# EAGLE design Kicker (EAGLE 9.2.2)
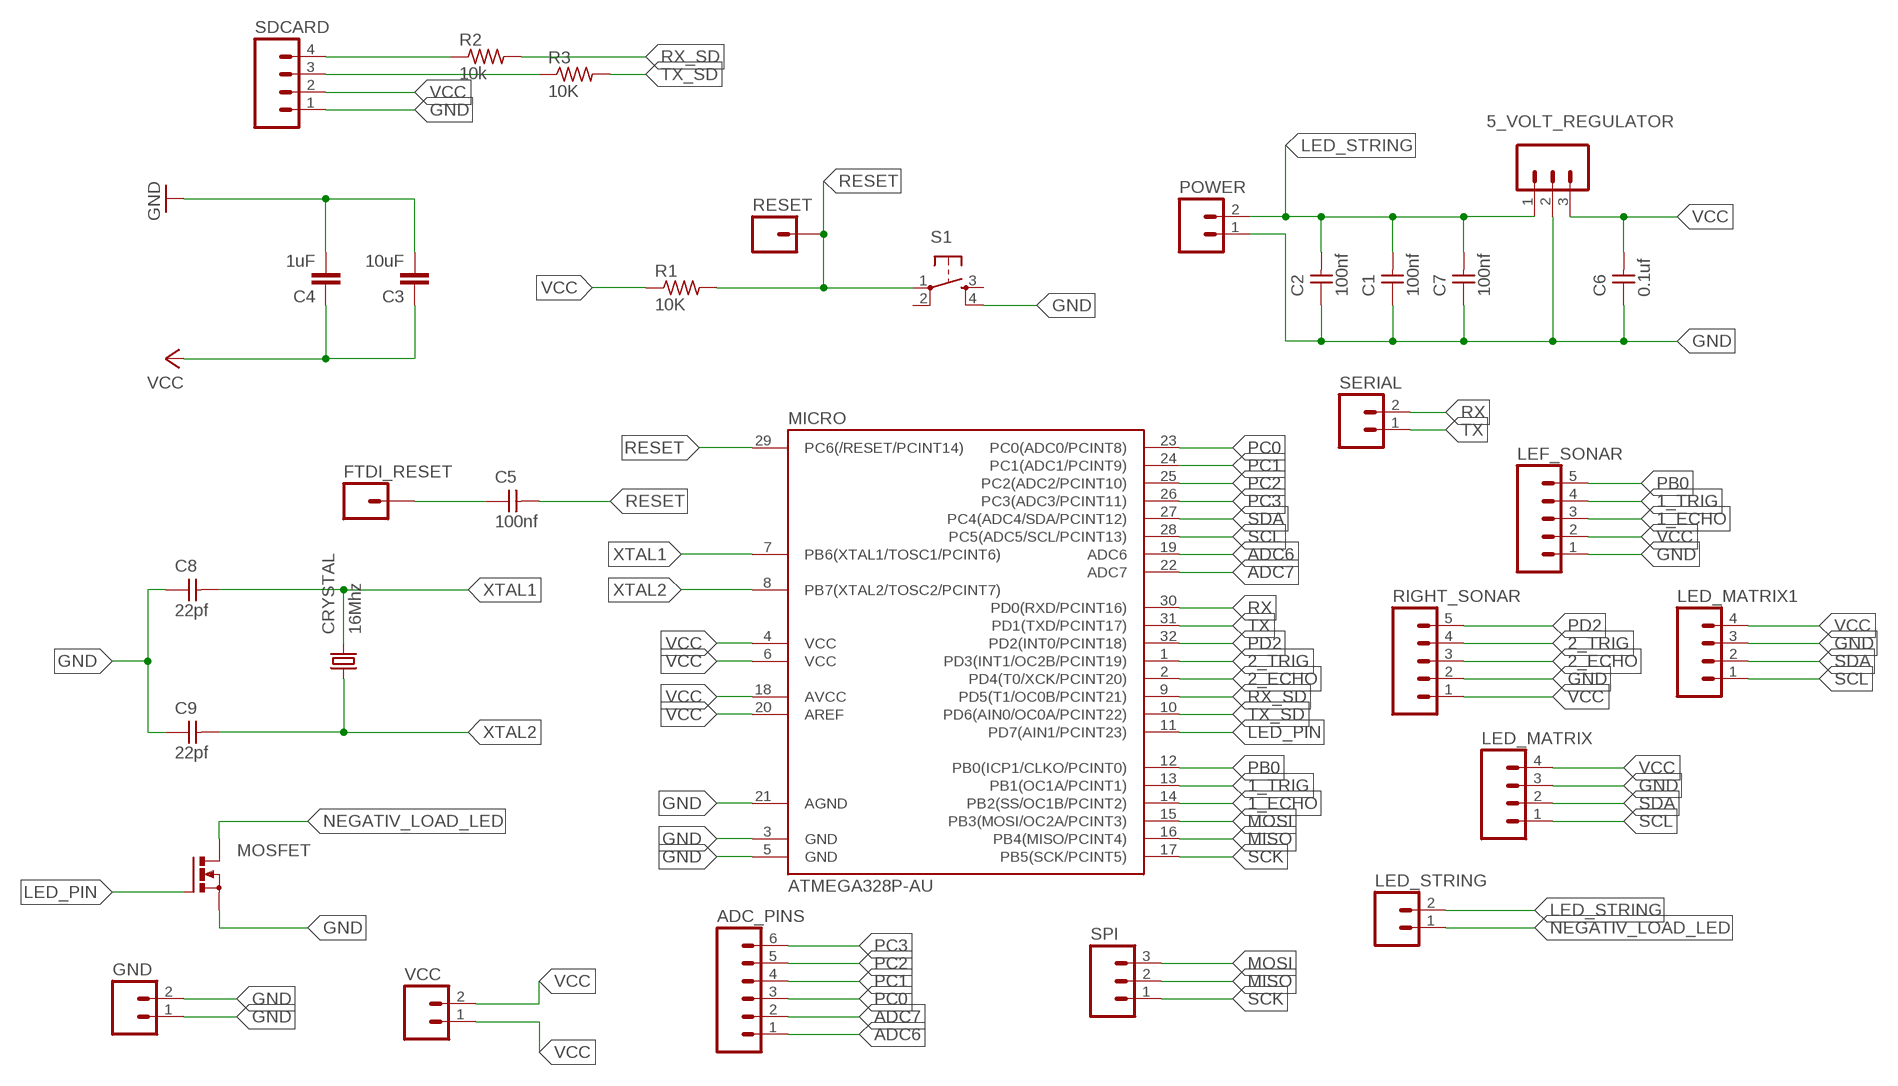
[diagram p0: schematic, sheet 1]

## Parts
5_VOLT_REGULATOR  M03  [03P]
ADC_PINS  M06  [06P]
C1  100nf  UNPOLARIZED_CAPACITOR1206  [1206]
C2  100nf  UNPOLARIZED_CAPACITOR1206  [1206]
C3  10uF  CAP1206  [1206]
C4  1uF  CAP1206  [1206]
C5  100nf  UNPOLARIZED_CAPACITOR1206  [1206]
C6  0.1uf  UNPOLARIZED_CAPACITOR1206  [1206]
C7  100nf  UNPOLARIZED_CAPACITOR1206  [1206]
C8  22pf  UNPOLARIZED_CAPACITOR1206  [1206]
C9  22pf  UNPOLARIZED_CAPACITOR1206  [1206]
CRYSTAL  16Mhz  KX-12B  [6.0X3.5_2]
FTDI_RESET  M01PTH  [1X01]
GND  M02  [02P]
LED_MATRIX  M04  [04P]
LED_MATRIX1  M04  [04P]
LED_STRING  M02  [02P]
LEF_SONAR  M05  [05P]
MICRO  ATMEGA328P-AU  ATMEGA48/88/168-AU  [TQFP32-08]
MOSFET  PMOSFET_NTO220BV  [TO220BV]
POWER  M02  [02P]
R1  10K  RESISTOR1206  [1206]
R2  10k  RESISTOR1206  [1206]
R3  10K  RESISTOR1206  [1206]
RESET  M01PTH  [1X01]
RIGHT_SONAR  M05  [05P]
S1  6MM_SWITCH6MM_SWITCH  [6MM_SWITCH]
SDCARD  M04  [04P]
SERIAL  M02  [02P]
SPI  M03  [03P]
VCC  M02  [02P]

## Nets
1_ECHO: LEF_SONAR.3 MICRO.14(PB2(SS/OC1B/PCINT2))
1_TRIG: LEF_SONAR.4 MICRO.13(PB1(OC1A/PCINT1))
2_ECHO: MICRO.2(PD4(T0/XCK/PCINT20)) RIGHT_SONAR.3
2_TRIG: MICRO.1(PD3(INT1/OC2B/PCINT19)) RIGHT_SONAR.4
ADC6: ADC_PINS.1 MICRO.19(ADC6)
ADC7: ADC_PINS.2 MICRO.22(ADC7)
GND: 5_VOLT_REGULATOR.2 C1.1 C2.1 C3.2 C4.2 C6.1 C7.1 C8.1 C9.1 GND.1 GND.2 LED_MATRIX1.3 LED_MATRIX.3 LEF_SONAR.1 MICRO.3(GND) MICRO.5(GND) MICRO.21(AGND) MOSFET.S POWER.1 RIGHT_SONAR.2 S1.4(S1) SDCARD.1
LED_PIN: MICRO.11(PD7(AIN1/PCINT23)) MOSFET.G
LED_STRING: 5_VOLT_REGULATOR.1 C1.2 C2.2 C7.2 LED_STRING.2 POWER.2
MISO: MICRO.16(PB4(MISO/PCINT4)) SPI.2
MOSI: MICRO.15(PB3(MOSI/OC2A/PCINT3)) SPI.3
N$2: R2.1 SDCARD.4
N$3: C5.1 FTDI_RESET.1
N$4: R3.1 SDCARD.3
NEGATIV_LOAD_LED: LED_STRING.1 MOSFET.D
PB0: LEF_SONAR.5 MICRO.12(PB0(ICP1/CLKO/PCINT0))
PC0: ADC_PINS.3 MICRO.23(PC0(ADC0/PCINT8))
PC1: ADC_PINS.4 MICRO.24(PC1(ADC1/PCINT9))
PC2: ADC_PINS.5 MICRO.25(PC2(ADC2/PCINT10))
PC3: ADC_PINS.6 MICRO.26(PC3(ADC3/PCINT11))
PD2: MICRO.32(PD2(INT0/PCINT18)) RIGHT_SONAR.5
RESET: C5.2 MICRO.29(PC6(/RESET/PCINT14)) R1.2 RESET.1 S1.1(P)
RX: MICRO.30(PD0(RXD/PCINT16)) SERIAL.2
RX_SD: MICRO.9(PD5(T1/OC0B/PCINT21)) R2.2
SCK: MICRO.17(PB5(SCK/PCINT5)) SPI.1
SCL: LED_MATRIX1.1 LED_MATRIX.1 MICRO.28(PC5(ADC5/SCL/PCINT13))
SDA: LED_MATRIX1.2 LED_MATRIX.2 MICRO.27(PC4(ADC4/SDA/PCINT12))
TX: MICRO.31(PD1(TXD/PCINT17)) SERIAL.1
TX_SD: MICRO.10(PD6(AIN0/OC0A/PCINT22)) R3.2
VCC: 5_VOLT_REGULATOR.3 C3.1 C4.1 C6.2 LED_MATRIX1.4 LED_MATRIX.4 LEF_SONAR.2 MICRO.4(VCC) MICRO.6(VCC) MICRO.18(AVCC) MICRO.20(AREF) R1.1 RIGHT_SONAR.1 SDCARD.2 VCC.1 VCC.2
XTAL1: C8.2 CRYSTAL.2 MICRO.7(PB6(XTAL1/TOSC1/PCINT6))
XTAL2: C9.2 CRYSTAL.1 MICRO.8(PB7(XTAL2/TOSC2/PCINT7))
Unconnected: S1.2(P1) S1.3(S)

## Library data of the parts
5_VOLT_REGULATOR SPI = con-amp-quick:M03: AMP QUICK CONNECTOR; OC_FARNELL: unknown; OC_NEWARK: unknown
ADC_PINS = con-amp-quick:M06: AMP QUICK CONNECTOR; OC_FARNELL: unknown; OC_NEWARK: unknown
C1 C2 C5-C9 = FAB_Hello:UNPOLARIZED_CAPACITOR: unpolarized_capacitor
C3 C4 = 01_SparkFun:CAP: Capacitor
CRYSTAL = crystal-geyer_V1_0:KX
FTDI_RESET RESET = flight_controller.lbr01_SparkFun:M01: Header 1
GND LED_STRING POWER SERIAL VCC = con-amp-quick:M02: AMP QUICK CONNECTOR; OC_FARNELL: unknown; OC_NEWARK: unknown
LED_MATRIX LED_MATRIX1 SDCARD = con-amp-quick:M04: AMP QUICK CONNECTOR; OC_FARNELL: unknown; OC_NEWARK: unknown
LEF_SONAR RIGHT_SONAR = con-amp-quick:M05: AMP QUICK CONNECTOR; OC_FARNELL: unknown; OC_NEWARK: unknown
MICRO = atmega8:ATMEGA48/88/168
MOSFET = transistor-power:PMOSFET_N: Power MOSFET N-Channel
R1-R3 = FAB_Hello:RESISTOR
S1 = FAB_Hello:6MM_SWITCH: OMRON SWITCH

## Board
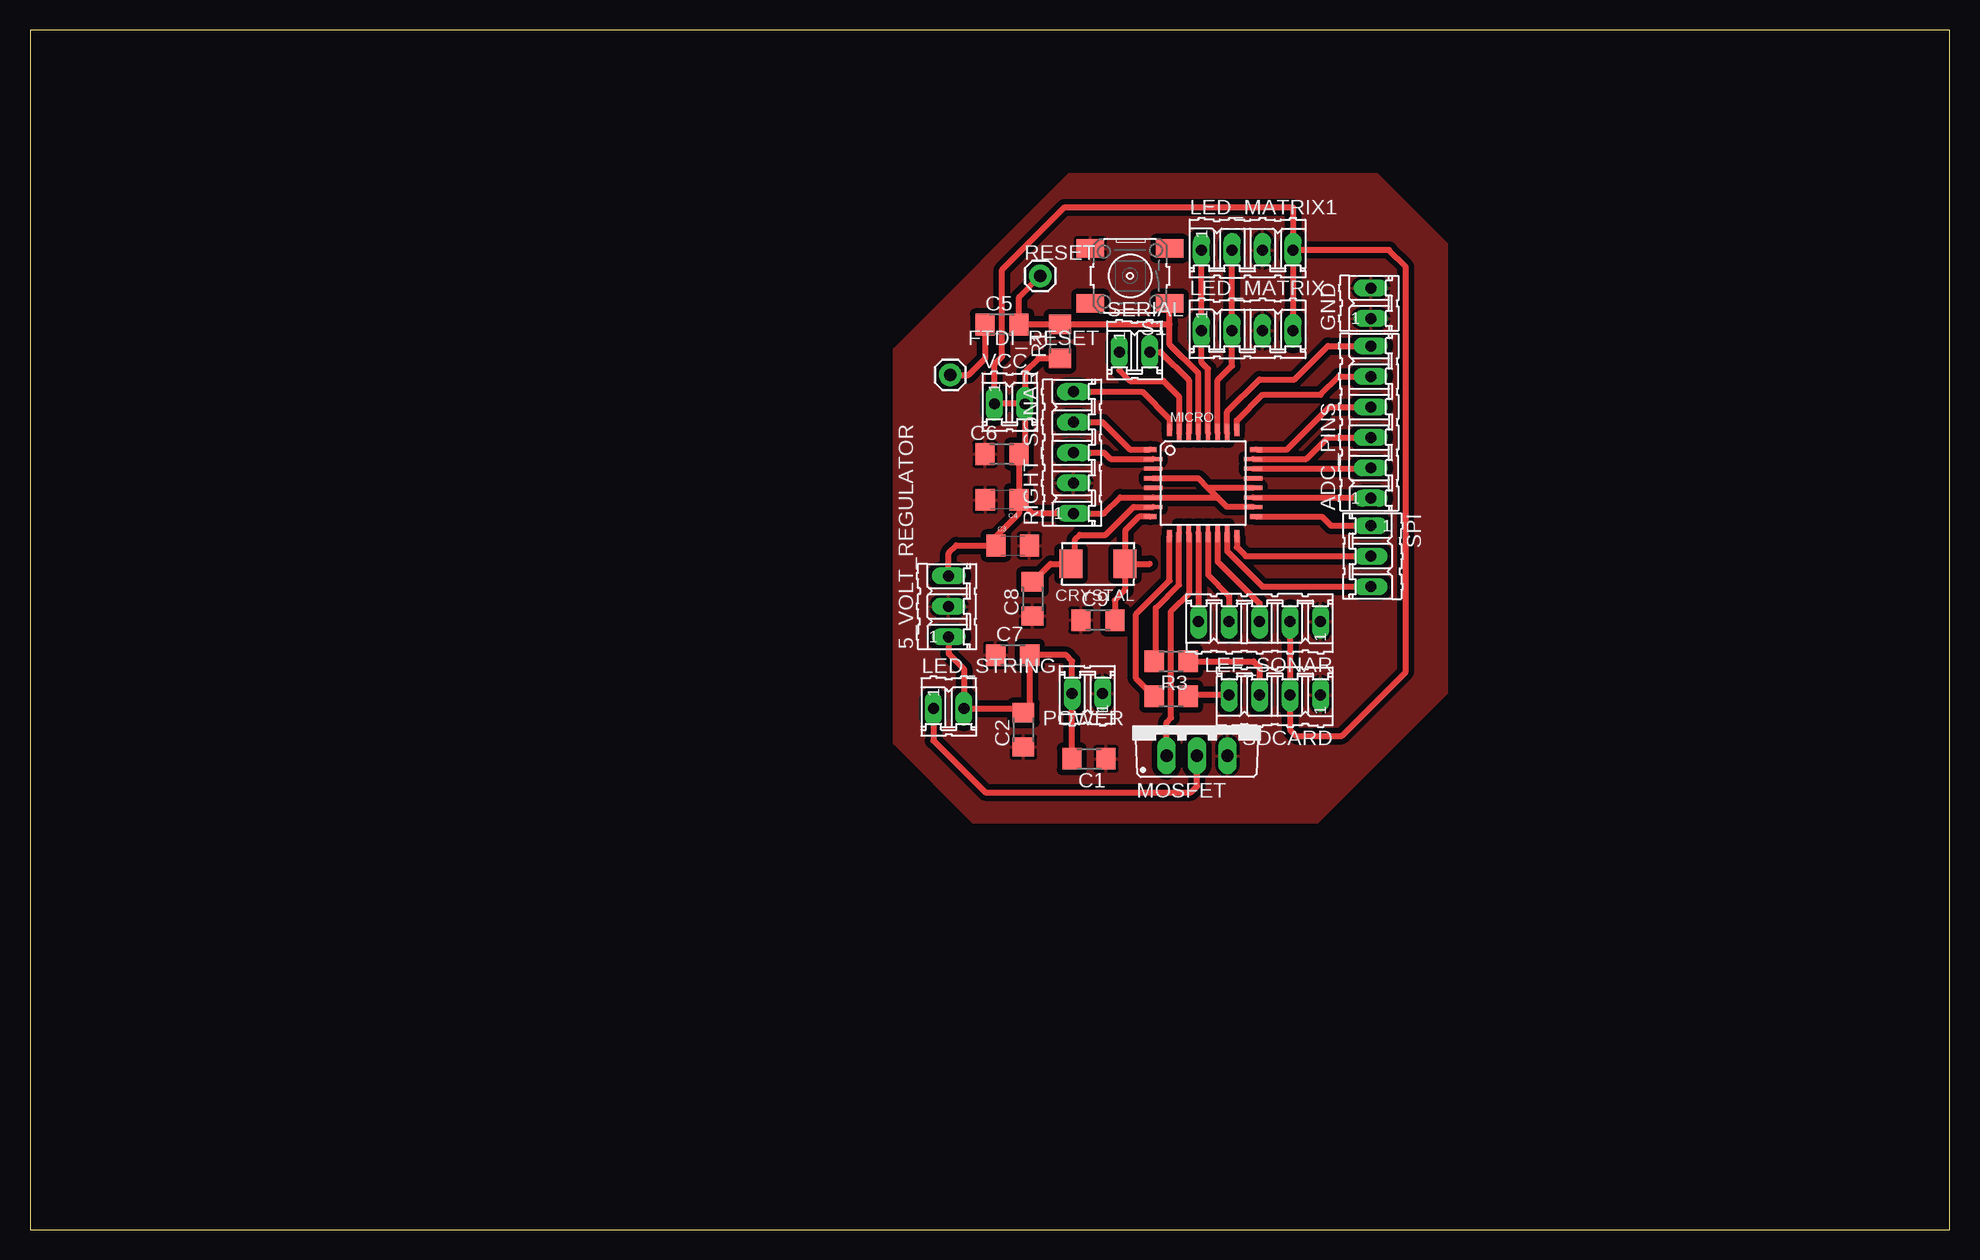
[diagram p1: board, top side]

Size 160 x 100 mm. Coordinates in mm from the lower left corner, seen from the top.
Outline: 0,0 160,0 160,100 0,100 0,0
Copper layers (1*16): Top 0.035mm / dielectric 1.5mm / Bottom 0.035mm
Design rules "default": minimum track width 6mil, minimum drill 0.35mm, track to track 6mil, track to pad 6mil, pad to pad 6mil, via to via 6mil, smd to smd 6mil, copper to edge 40mil, drill to drill 6mil, minimum pad ring 10mil, minimum via ring 8mil, stop-mask expansion 4mil, vias tented up to drill 0mil, thermal gap 10mil

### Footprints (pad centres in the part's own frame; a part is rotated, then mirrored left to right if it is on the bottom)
03P = drill 0.914 long: 1 -2.54,0; 2 0,0; 3 2.54,0
06P = drill 0.914 long: 1 -6.35,0; 2 -3.81,0; 3 -1.27,0; 4 1.27,0; 5 3.81,0; 6 6.35,0
1206 = smd 1.6 x 1.803: 1 -1.422,0; 2 1.422,0
1206' = smd 1.6 x 1.8: 1 -1.4,0; 2 1.4,0
6.0X3.5_2 = smd 1.9 x 2.4: 1 -2.25,0; 2 2.25,0
1X01 = drill 1.016 pad 1.88: 1 0,0
02P = drill 0.914 long: 1 -1.27,0; 2 1.27,0
04P = drill 0.914 long: 1 -3.81,0; 2 -1.27,0; 3 1.27,0; 4 3.81,0
05P = drill 0.914 long: 1 -5.08,0; 2 -2.54,0; 3 0,0; 4 2.54,0; 5 5.08,0
TQFP32-08 = smd 1.016 x 0.406: 1 -4.42,2.8; 8 -4.42,-2.8; 17 4.42,-2.8; 24 4.42,2.8 | smd 1.524 x 0.356: 2 -4.166,2; 3 -4.166,1.2; 4 -4.166,0.4; 5 -4.166,-0.4; 6 -4.166,-1.2; 7 -4.166,-2; 18 4.166,-2; 19 4.166,-1.2; 20 4.166,-0.4; 21 4.166,0.4; 22 4.166,1.2; 23 4.166,2 | smd 0.406 x 1.016: 9 -2.8,-4.42; 16 2.8,-4.42; 25 2.8,4.42; 32 -2.8,4.42 | smd 0.356 x 1.524: 10 -2,-4.166; 11 -1.2,-4.166; 12 -0.4,-4.166; 13 0.4,-4.166; 14 1.2,-4.166; 15 2,-4.166; 26 2,4.166; 27 1.2,4.166; 28 0.4,4.166; 29 -0.4,4.166; 30 -1.2,4.166; 31 -2,4.166
TO220BV = drill 1.016 long: D 0,-2.54; G -2.54,-2.54; S 2.54,-2.54
6MM_SWITCH = smd 2.286 x 1.524: 1 -3.302,2.286; 2 3.302,2.286; 3 -3.302,-2.286; 4 3.302,-2.286

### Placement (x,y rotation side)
5_VOLT_REGULATOR  76.58,51.94 90 top
ADC_PINS  111.76,67.31 90 top
C1  88.27,39.24 180 top
C2  82.8,41.66 90 top
C3  10uF  [1206']  81.92,57.02 0 top
C4  1uF  [1206']  81.03,60.83 180 top
C5  81.03,75.44 0 top
C6  81.03,64.64 0 top
C7  81.92,47.88 0 top
C8  83.57,52.58 90 top
C9  89.03,50.8 0 top
CRYSTAL  89.03,55.5 180 top
FTDI_RESET  76.71,71.25 0 top
GND  111.76,77.22 90 top
LED_MATRIX  101.47,74.93 0 top
LED_MATRIX1  101.47,81.66 0 top
LED_STRING  76.58,43.43 0 top
LEF_SONAR  102.49,50.67 180 top
MICRO  97.79,62.23 0 top
MOSFET  97.28,42.04 0 top
POWER  88.14,44.7 180 top
R1  85.85,74.04 90 top
R2  95.12,44.45 180 top
R3  95.12,47.37 180 top
RESET  84.2,79.5 0 top
RIGHT_SONAR  87,64.77 90 top
S1  91.69,79.5 180 top
SDCARD  103.76,44.58 180 top
SERIAL  92.08,73.15 0 top
SPI  111.76,56.13 270 top
VCC  81.66,68.83 0 top

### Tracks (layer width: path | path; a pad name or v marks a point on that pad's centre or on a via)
1_ECHO
  Top 0.508: MICRO.14 98.99,55.7 102.49,52.2 LEF_SONAR.3
1_TRIG
  Top 0.508: MICRO.13 98.19,54.59 99.95,52.83 LEF_SONAR.4
2_ECHO
  Top 0.508: RIGHT_SONAR.3 89.53,64.77 90.08,64.23 MICRO.2
2_TRIG
  Top 0.508: RIGHT_SONAR.4 89.41,67.31 91.69,65.02 MICRO.1
ADC6
  Top 0.508: MICRO.19 111.69,61.03 ADC_PINS.1
ADC7
  Top 0.508: MICRO.22 111.69,63.43 ADC_PINS.2
GND
  pour Top (isolate 0.457): 86.61,88.01 112.27,88.01 118.11,82.17 118.11,44.7 107.31,33.91 78.61,33.91 72.01,40.51 72.01,73.41
LED_PIN
  Top 0.508: MICRO.11 96.59,53.03 95.12,51.56 95.12,42.67 94.74,42.29 MOSFET.G
LED_STRING
  Top 0.508: C1.2 86.84,44.68 POWER.2 86.87,47.37 86.36,47.88 C7.2 83.34,43.61 C2.2 82.45,43.43 LED_STRING.2 77.85,46.74 76.58,48.01 5_VOLT_REGULATOR.1
MISO
  Top 0.508: MICRO.16 100.59,56.89 101.35,56.13 SPI.2
MOSI
  Top 0.508: MICRO.15 99.79,56.55 102.74,53.59 SPI.3
N$2
  Top 0.508: SDCARD.4 96.67,44.58 R2.1
N$3
  Top 0.508: FTDI_RESET.1 78.23,71.25 79.63,72.64 79.63,75.41 C5.1
N$4
  Top 0.508: R3.1 101.98,47.37 102.49,46.86 SDCARD.3
NEGATIV_LOAD_LED
  Top 0.508: LED_STRING.1 75.31,40.77 79.63,36.45 96.77,36.45 97.28,36.96 MOSFET.D
PB0
  Top 0.508: MICRO.12 97.41,58.05 LEF_SONAR.5
PC0
  Top 0.508: MICRO.23 106.39,64.23 108.2,66.04 ADC_PINS.3
PC1
  Top 0.508: MICRO.24 104.78,65.03 108.33,68.58 ADC_PINS.4
PC2
  Top 0.508: MICRO.25 100.59,67.44 102.74,69.6 107.57,69.6 109.09,71.12 ADC_PINS.5
PC3
  Top 0.508: MICRO.26 99.79,68.17 102.49,70.87 105.41,70.87 108.2,73.66 ADC_PINS.6
PD2
  Top 0.508: RIGHT_SONAR.5 92.71,69.85 95,67.56 94.99,67.56 MICRO.32
RESET
  Top 0.508: MICRO.29 97.39,71.39 95,73.79 95,75.44 | 95,75.44 S1.1 | 95,75.44 94.97,75.46 R1.2 85.83,75.44 C5.2 82.45,77.75 RESET.1
RX
  Top 0.508: SERIAL.2 94.23,73.15 96.59,70.8 MICRO.30
RX_SD
  Top 0.508: R2.2 92.2,45.95 92.2,51.31 94.99,54.1 MICRO.9
SCK
  Top 0.508: MICRO.17 107.7,59.43 108.46,58.67 SPI.1
SCL
  Top 0.508: MICRO.28 98.19,71.74 97.66,72.26 LED_MATRIX.1 LED_MATRIX1.1
SDA
  Top 0.508: MICRO.27 98.99,70.8 100.2,72.01 LED_MATRIX.2 LED_MATRIX1.2
TX
  Top 0.508: SERIAL.1 90.81,71.63 91.69,70.74 94.49,70.74 95.79,69.44 MICRO.31
TX_SD
  Top 0.508: R3.2 93.85,47.52 93.85,51.82 95.79,53.75 MICRO.10
VCC
  Top 0.508: MICRO.4 97.39,62.63 98.19,61.83 | MICRO.18 99.79,60.23 98.99,61.03 | 98.99,61.03 98.19,61.83 | 98.99,61.03 MICRO.6 90.88,61.03 89.53,59.69 RIGHT_SONAR.1 83.57,59.69 C4.1 | LEF_SONAR.2 SDCARD.2 105.03,41.66 105.54,41.15 109.35,41.15 114.68,46.48 114.68,80.26 113.28,81.66 LED_MATRIX1.4 | R1.1 84.05,72.62 82.93,71.5 VCC.2 | VCC.2 VCC.1 80.39,72.14 81.03,72.77 81.03,80.01 86.23,85.22 105.28,85.22 LED_MATRIX1.4 | VCC.2 82.93,65.13 C6.2 82.45,60.85 C4.1 | C4.1 82.43,59.69 80.52,57.78 C3.1 77.22,57.02 76.58,56.39 5_VOLT_REGULATOR.3 | LED_MATRIX1.4 LED_MATRIX.4 | MICRO.20 98.19,61.83
XTAL1
  Top 0.508: C8.2 85.06,55.5 CRYSTAL.2 87.12,55.84 87.12,57.53 87.5,57.91 89.66,57.91 91.98,60.23 MICRO.7
XTAL2
  Top 0.508: 90.77,51.12 C9.2 90.42,50.83 90.42,52.45 91.28,53.3 CRYSTAL.1 | MICRO.8 92.45,59.43 91.28,58.26 CRYSTAL.1 | CRYSTAL.1 93.34,55.5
